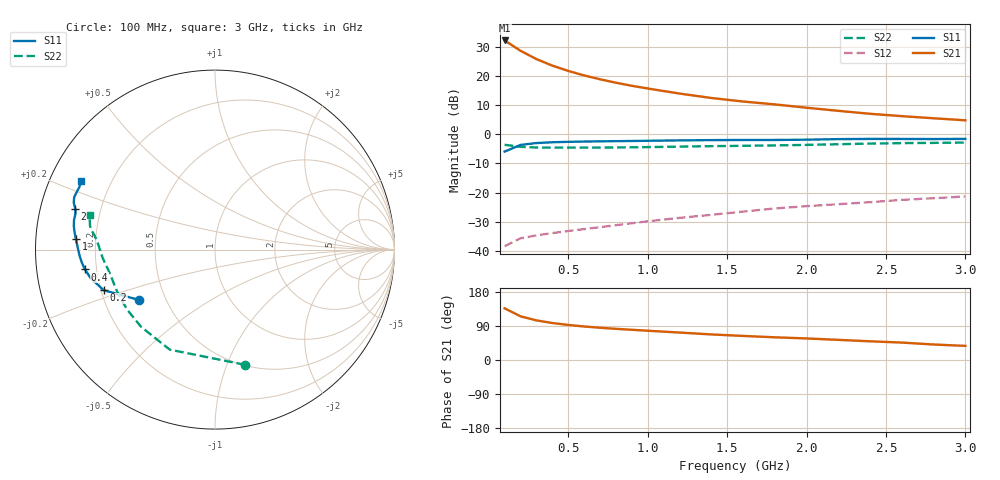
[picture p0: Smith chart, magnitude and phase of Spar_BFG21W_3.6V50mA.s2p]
! Filename: 3_650bfg21.001
! Title: BFG21W
! Bias: Vce=3.6V; Ic=50mA
! Company: NXP Semiconductors NL
! User: Quality&Reliability T&D
! Measure time: 10 Nov 1999 / 11:43:58
#  MHz  S  MA  R 50
! Freq  S11  S21  S12  S22  :
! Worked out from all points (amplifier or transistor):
!   20 points, 100 MHz to 3 GHz, reference 50 ohm
!   highest |S21| = 32.4 dB at 100 MHz (marker M1)
!   |S21| within 3 dB of that: start of sweep to 184.6 MHz
!   unconditionally stable (mu >= 1): 866.5 MHz to end of sweep
!   at 400 MHz: K = 0.70, MSG = 28.8 dB, |S12| = -34.0 dB
!   at 1.2 GHz: K = 1.07, MAG = 19.8 dB, |S12| = -28.7 dB
!   at 3 GHz: K = 1.05, MAG = 11.7 dB, |S12| = -21.4 dB
!   S11 on the Smith chart (normalised r, x): 100 MHz: 0.35, -0.27; 200 MHz: 0.21, -0.17; 400 MHz: 0.16, -0.07; 1 GHz: 0.13, +0.04; 2 GHz: 0.11, +0.14; 3 GHz: 0.09, +0.24
100  0.5066 -146.3  41.45 136.3  0.01192 48.8  0.6631 -75.4
200  0.6596 -159.9  27.56 115.3  0.01622 41.5  0.6117 -114.3
300  0.7103 -167.0  19.82 104.6  0.01831 41.1  0.5956 -133.7
400  0.7329 -171.3  15.3 97.7  0.02 43.4  0.5923 -144.8
500  0.7457 -174.5  12.41 92.5  0.0217 46.0  0.5923 -152.0
600  0.7539 -177.0  10.37 88.5  0.02341 49.0  0.5931 -157.0
700  0.7598 -179.1  8.906 85.1  0.02532 51.9  0.5942 -160.8
800  0.7654 179.0  7.772 82.2  0.02738 54.5  0.5962 -163.9
900  0.7712 177.3  6.882 79.8  0.02956 57.2  0.6 -166.6
1000  0.7777 175.7  6.175 77.3  0.03193 59.1  0.6048 -169.0
1200  0.7891 172.8  5.058 72.5  0.03659 62.3  0.6167 -172.8
1400  0.7977 170.5  4.241 67.5  0.04129 64.4  0.6283 -176.0
1600  0.8025 168.2  3.687 63.5  0.04692 66.2  0.6364 -178.6
1800  0.8028 165.6  3.286 59.9  0.05311 67.4  0.6465 178.6
2000  0.8118 163.7  2.882 56.9  0.05822 68.9  0.6602 175.6
2200  0.8297 161.6  2.547 53.1  0.0629 69.4  0.6775 173.1
2400  0.8367 159.7  2.264 49.3  0.06812 69.2  0.6957 171.2
2600  0.8352 157.8  2.064 46.0  0.07468 68.7  0.7079 169.5
2800  0.832 155.4  1.896 40.9  0.07971 67.4  0.7149 167.3
3000  0.8378 152.8  1.749 37.3  0.0856 66.8  0.7241 164.7
